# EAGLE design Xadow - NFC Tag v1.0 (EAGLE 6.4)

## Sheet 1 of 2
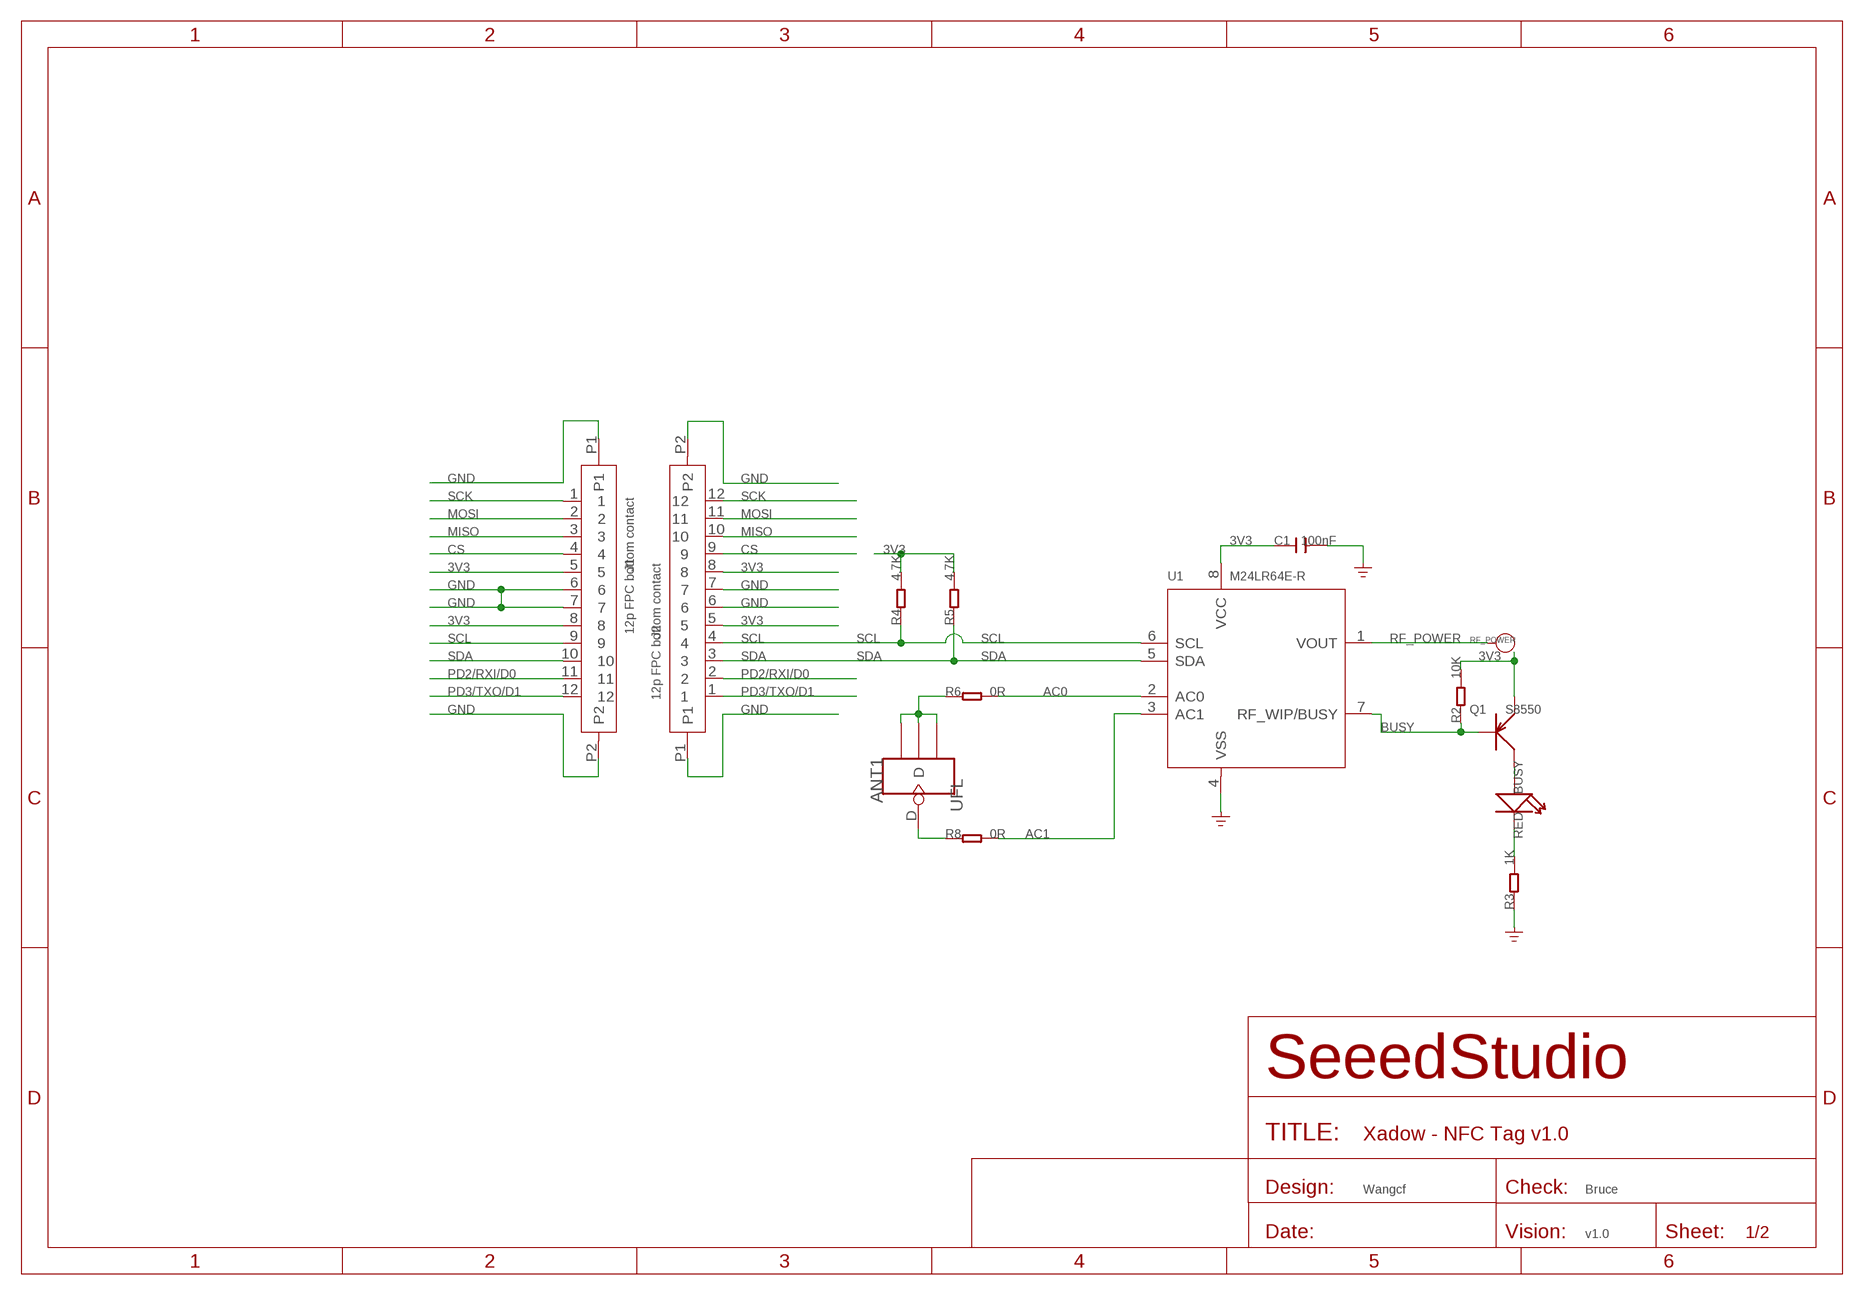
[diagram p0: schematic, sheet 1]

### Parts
ANT1  UFL  ANTENNA-U-FL  [4P-U-FL]
BUSY  RED  LED'0603'  [LED-0603]
C1  100nF  C-0402  [C0402]
J1  12p FPC bottom contact  FPC052002-12LT-FH12-12S-0.5SH  [12P-0.5-NEW]
J2  12p FPC bottom contact  FPC052002-12LT-FH12-12S-0.5SH  [12P-0.5-NEW]
Q1  S8550  TRANSISTOR-PNP-SOT23  [SOT23]
R2  10K  R-0402  [R0402]
R3  1K  R-0402  [R0402]
R4  4.7K  R-0402  [R0402]
R5  4.7K  R-0402  [R0402]
R6  0R  R-0402  [R0402]
R8  0R  R-0402  [R0402]
RF_POWER  PAD-TEST-POINT'4545'  [TP_4545]
U1  M24LR64E-R  [TSSOP8]

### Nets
3V3: C1.1 J1.5 J1.8 J2.5 J2.8 Q1.2(E) R2.2 R4.2 R5.2 U1.8(VCC)
AC0: R6.2 U1.2(AC0)
AC1: R8.2 U1.3(AC1)
BUSY: Q1.1(B) R2.1 U1.7(RF_WIP/BUSY)
CS: J1.4 J2.9
GND: C1.2 J1.6 J1.7 J1.P1 J1.P2 J2.6 J2.7 J2.P1 J2.P2 R3.1 U1.4(VSS)
MISO: J1.3 J2.10
MOSI: J1.2 J2.11
N$3: BUSY.+ Q1.3(C)
N$9: BUSY.- R3.2
N$17: ANT1.D R8.1
N$18: ANT1.GND1 ANT1.GND2 ANT1.GND3 R6.1
PD2/RXI/D0: J1.11 J2.2
PD3/TXO/D1: J1.12 J2.1
RF_POWER: RF_POWER.T U1.1(VOUT)
SCK: J1.1 J2.12
SCL: J1.9 J2.4 R4.1 U1.6(SCL)
SDA: J1.10 J2.3 R5.1 U1.5(SDA)

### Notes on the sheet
- Wangcf | Bruce
- v1.0

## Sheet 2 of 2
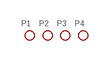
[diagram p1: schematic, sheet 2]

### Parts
P1  PAD-MARK  [ROUND-MARK-1.0]
P2  PAD-MARK  [ROUND-MARK-1.0]
P3  PAD-MARK  [ROUND-MARK-1.0]
P4  PAD-MARK  [ROUND-MARK-1.0]

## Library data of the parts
ANT1 = Connector:ANTENNA-U-FL
BUSY = Discrete:LED*
C1 = Discrete:C*: Ceramic Capacitors
J1 J2 = template :FPC052002-12LT
P1-P4 = Discrete:PAD-MARK; PARTNO: DNP
Q1 = Discrete:TRANSISTOR-PNP*: PNP audion
R2-R6 R8 = Discrete:R*
RF_POWER = Discrete:PAD-TEST-POINT; PARTNO: DNP
U1 = template:M24LR64E-R: Dynamic NFC/RFID tag IC with 64-Kbit EEPROM, energy harvesting, I²C bus and ISO 15693 RF interface

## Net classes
0 default: width 0.152 mm, drill 0.305 mm, clearance 0.152 mm
1 GND: width 0.152 mm, drill 0.305 mm, clearance 0.152 mm to class 0, clearance 0.152 mm
3 usbvcc: width 0.203 mm, drill 0.305 mm, clearance 0.203 mm

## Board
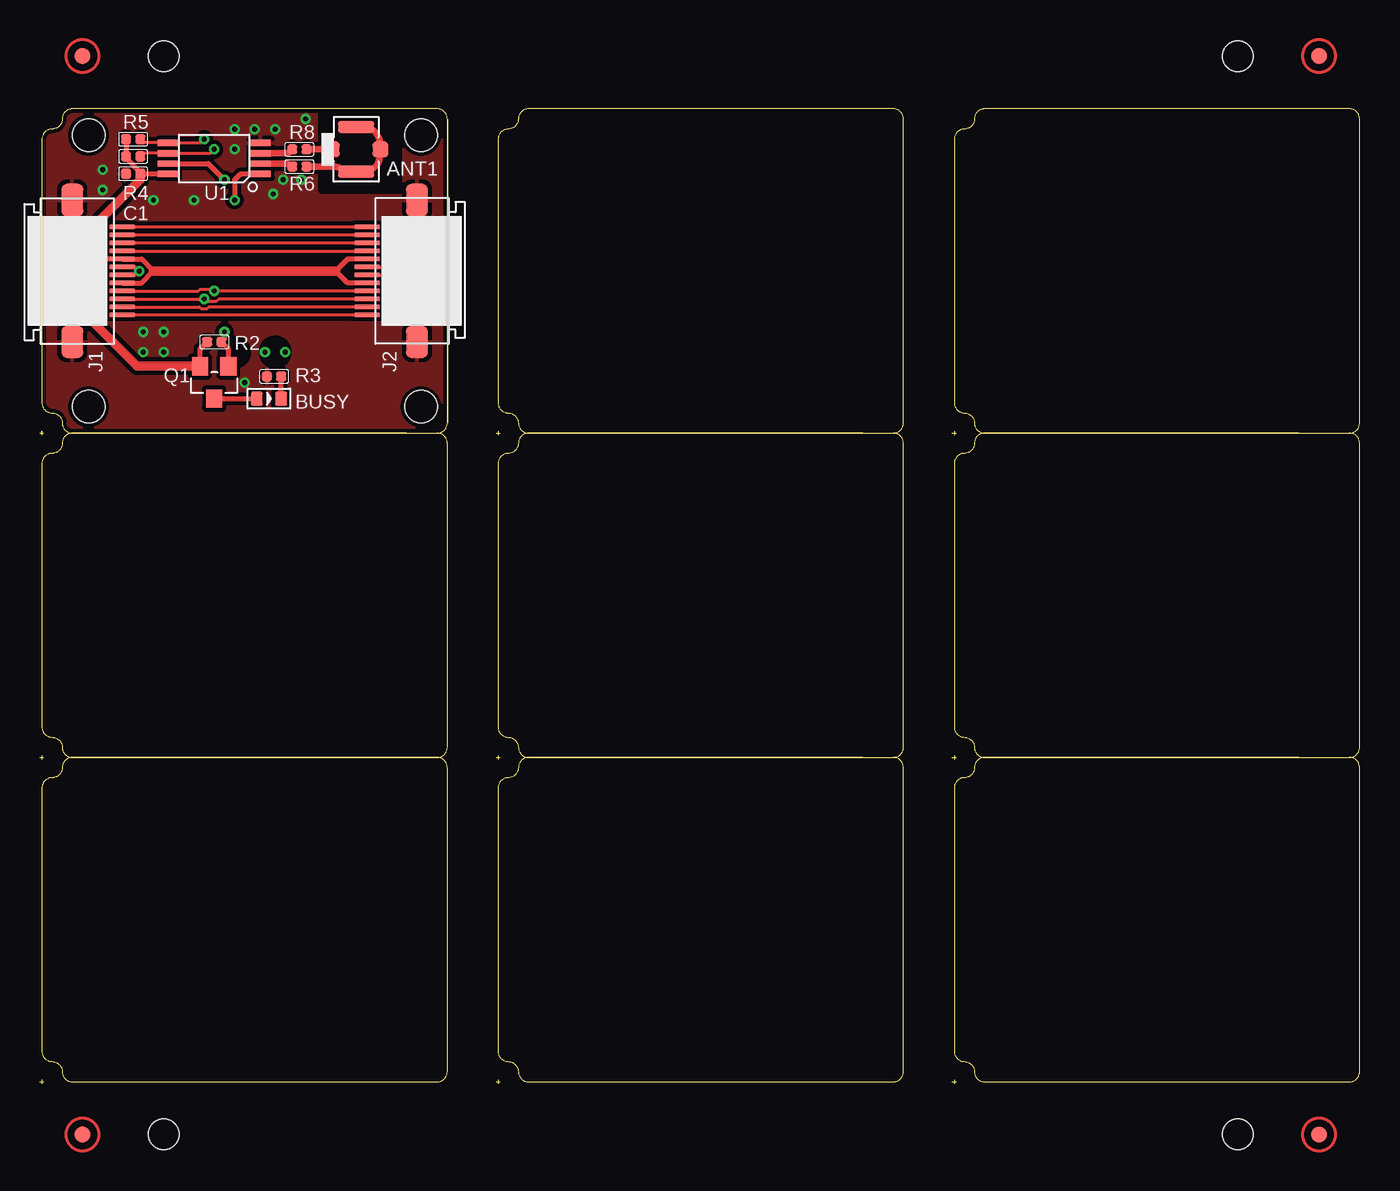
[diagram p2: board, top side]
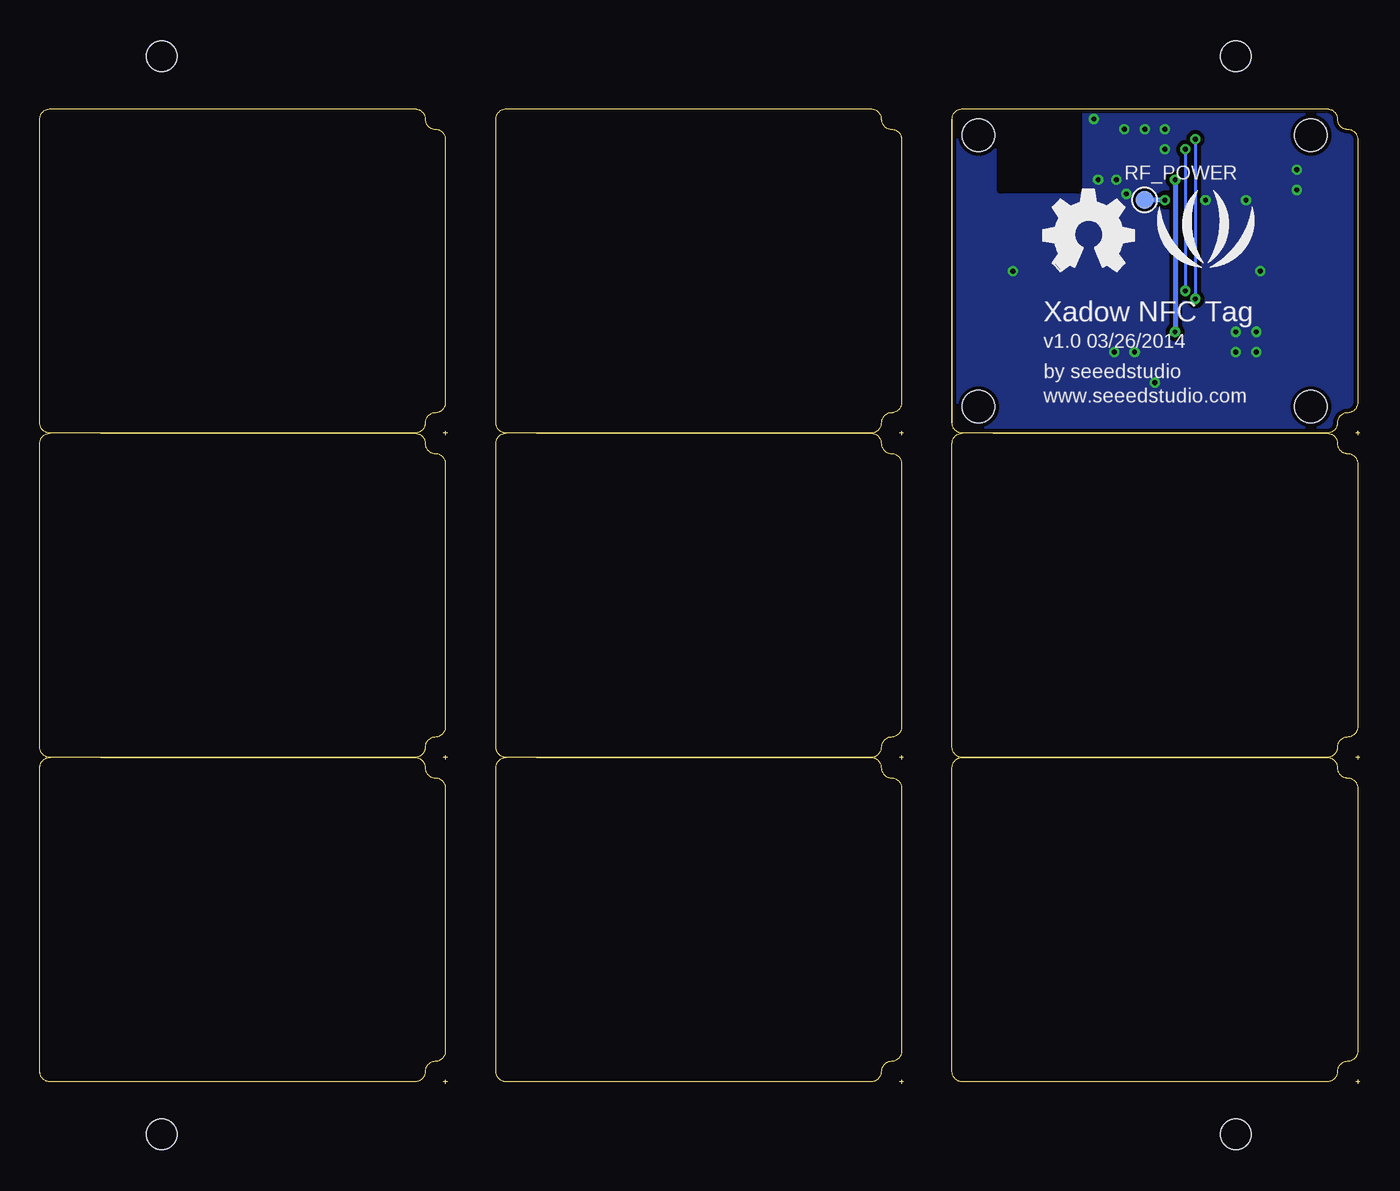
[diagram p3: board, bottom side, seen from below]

Size 82.68 x 61.09 mm. Coordinates in mm from the lower left corner, seen from the top.
Outline: 168 segments
Copper layers (1*16): Top 0.035mm / dielectric 1.5mm / Bottom 0.035mm
Design rules "SeeedStudio_2layer_DRU_no_angle_20140221 *": minimum track width 6mil, minimum drill 12mil, track to track 6mil, track to pad 6mil, pad to pad 6mil, via to via 6mil, smd to smd 0mil, copper to edge 10mil, drill to drill 10mil, minimum pad ring 10mil, minimum via ring 6mil, stop-mask expansion 2mil, vias tented up to drill 100mil, thermal gap 10mil
Holes 2.03 mm at 3.05,42.42 3.05,59.44 23.88,59.44 23.88,42.42
Holes 1.91 mm at 75.06,64.39 7.75,64.39 7.75,-3.17 75.06,-3.17
tRestrict: area 17.7,56 to 22.5,61.2; area 4.6,50.9 to 5.2,51; area 20.4,50.9 to 21,51; area 11.2,50 to 12.1,50.2; area 11.6,45.2 to 12.8,46.5; area 14.1,45.2 to 15.4,46.5; 13 lines
bRestrict: area 17.7,56 to 22.5,61.2; 13 lines

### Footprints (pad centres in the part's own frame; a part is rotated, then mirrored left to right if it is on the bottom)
4P-U-FL = smd 1.016 x 1.016: D -1.524,0; GND3 1.524,0 | smd 2.286 x 0.762: GND1 0,1.397; GND2 0,-1.397
LED-0603 = smd 0.762 x 0.889: + -0.762,0; - 0.762,0
C0402 = smd 0.635 x 0.635: 1 -0.445,0; 2 0.445,0
12P-0.5-NEW = smd 0.3 x 1.6: 1 -2.75,3.127; 2 -2.25,3.127; 3 -1.75,3.127; 4 -1.25,3.127; 5 -0.75,3.127; 6 -0.25,3.127; 7 0.25,3.127; 8 0.75,3.127; 9 1.25,3.127; 10 1.75,3.127; 11 2.25,3.127; 12 2.75,3.127 | smd 2.032 x 1.397: P1 -4.445,0; P2 4.445,0
ROUND-MARK-1.0 = smd 1.016 x 1.016: P$1 0,0
SOT23 = smd 1.016 x 1.143: 1 -0.889,-1.016; 2 0.889,-1.016; 3 0,1.016
R0402 = smd 0.635 x 0.635: 1 -0.445,0; 2 0.445,0
TP_4545 = smd 1.143 x 1.143: T 0,0
TSSOP8 = smd 0.4 x 1.27: 1 -0.975,-2.9; 2 -0.325,-2.9; 3 0.325,-2.9; 4 0.975,-2.9; 5 0.975,2.9; 6 0.325,2.9; 7 -0.325,2.9; 8 -0.975,2.9

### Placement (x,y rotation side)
ANT1  19.81,58.55 0 top
BUSY  14.35,42.93 0 top
C1  5.84,57.02 180 top
J1  2.03,50.93 270 top
J2  23.62,50.93 90 top
P1  not placed on the board
P2  not placed on the board
P3  not placed on the board
P4  not placed on the board
Q1  10.92,43.94 180 top
R2  10.92,46.48 180 top
R3  14.67,44.32 0 top
R4  5.84,58.1 180 top
R5  5.84,59.18 180 top
R6  16.26,57.47 180 top
R8  16.26,58.55 180 top
RF_POWER  13.46,55.37 0 bottom
U1  10.92,57.98 90 top
U$2  [OSHW_FILLX200_NOTEXT]  19.81,50.93 0 bottom
U$3  [LOGO_SILK]  9.65,52.83 0 bottom

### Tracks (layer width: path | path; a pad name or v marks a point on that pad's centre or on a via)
3V3
  Top 0.305: U1.8 6.31,57 C1.1 6.29,57.12 5.4,58.01 R4.2 R5.2 | Q1.2 10.03,46.04 R2.2 | J1.8 6.36,50.18 7.11,50.93 6.36,51.68 J1.5 3.7,51.68 | J2.8 19.29,51.68 18.54,50.93 19.29,50.18 J2.5 | 3.67,51.68 3.44,51.68 3.3,51.82 | 3.7,51.68 3.67,51.68 | 3.67,51.68 3.43,51.44 | 3.7,51.68 3.43,51.94
  Top 0.61: 18.54,50.93 7.11,50.93 | C1.1 6.29,56.64 3.3,53.66 3.3,51.82 3.3,47.75 6.1,44.96 Q1.2
AC0
  Top 0.406: U1.2 15.37,57.65 arc-45 R6.2
AC1
  Top 0.406: U1.3 15.39,58.3 arc45 15.69,58.42 R8.2
BUSY  (via drill 0.3 pad 0.64)
  Top 0.305: Q1.1 11.81,46.04 R2.1 | U1.7 10.55,57.65 v11.56,56.64 | 11.49,46.61 R2.1 | v11.56,47.12 11.56,46.67 R2.1
  Bottom 0.305: v11.56,56.64 v11.56,47.12
CS
  Top 0.203: J1.4 J2.9
GND  (via drill 0.3 pad 0.64)
  Top 0.203: J2.7 21.47,51.18 v21.72,50.93 21.47,50.68 J2.6 | J1.6 5.97,51.18 v6.22,50.93 5.97,50.68 J1.7
  other vias: 6.48,47.12 7.75,47.12 7.75,45.85 6.48,45.85 3.94,57.28 3.94,56.01 12.19,58.55 12.19,59.82 13.46,59.82 14.73,59.82 12.83,43.94 14.1,45.85 15.37,45.85 7.11,55.37 9.65,55.37 16.64,60.45 14.61,55.75 16.38,56.64 15.24,56.64
  pour Top (isolate 0.254): 0.13,61.09 25.53,61.09 25.53,40.77 0.13,40.77
  pour Bottom (isolate 0.254): 0.13,61.09 25.53,61.09 25.53,40.77 0.13,40.77
MISO
  Top 0.203: J2.10 J1.3
MOSI
  Top 0.203: J2.11 J1.2
N$3
  Top 0.305: Q1.3 BUSY.+
N$9
  Top 0.305: BUSY.- R3.2
N$17
  Top 0.406: R8.1 ANT1.D
N$18
  Top 0.406: ANT1.GND1 20.7,59.94 20.96,59.68 arc-45 21.34,58.78 ANT1.GND3 21.34,58.28 arc-45 20.98,57.43 20.7,57.15 ANT1.GND2 19.05,57.15 18.97,57.23 arc45 18.4,57.47 R6.1
PD2/RXI/D0
  Top 0.203: J1.11 10,48.68 10.11,48.57 10.47,48.57 10.58,48.68 J2.2
PD3/TXO/D1
  Top 0.203: J2.1 J1.12
RF_POWER  (via drill 0.3 pad 0.64)
  Top 0.305: U1.1 12.55,57 12.19,56.64 v12.19,55.37
  Bottom 0.305: v12.19,55.37 RF_POWER.T
SCK
  Top 0.203: J2.12 J1.1
SCL  (via drill 0.3 pad 0.64)
  Top 0.203: R4.1 6.48,58.3 U1.6 10.68,58.3 v10.92,58.55 | J1.9 9.93,49.68 10.03,49.78 10.81,49.78 v10.92,49.68 J2.4
  Bottom 0.203: v10.92,58.55 v10.92,49.68
SDA  (via drill 0.3 pad 0.64)
  Top 0.203: J1.10 v10.29,49.18 10.39,49.18 10.53,49.04 11.06,49.04 11.2,49.18 J2.3 | R5.1 6.52,58.95 U1.5 10.05,58.95 v10.29,59.18
  Bottom 0.203: v10.29,59.18 v10.29,49.18

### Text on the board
bPlace: Xadow NFC Tag | v1.0 03/26/2014 | by seeedstudio | www.seeedstudio.com
tEnhance: Top Enhance 0.25~0.28mm
bEnhance: Bottom Enhance
bEnHoles: Holes on Bottom Enhance | All Holes are 70mil diameter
